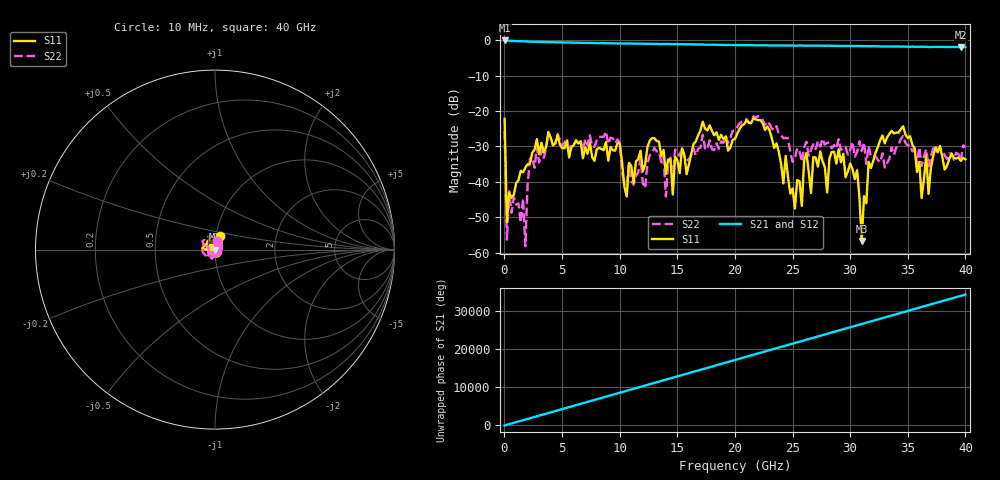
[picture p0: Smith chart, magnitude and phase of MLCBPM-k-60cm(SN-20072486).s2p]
!Keysight Technologies,N5225A,MY51451228,A.10.40.14
!Date: Friday, November 20, 2020 11:33:09
!Correction: S11(Full 2 Port(1,2))
!S21(Full 2 Port(1,2))
!S12(Full 2 Port(1,2))
!S22(Full 2 Port(1,2))
!S2P File: Measurements: S11, S21, S12, S22:
# Hz S  dB  R 50
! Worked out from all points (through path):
!   201 points, 10 MHz to 40 GHz, reference 50 ohm
!   highest |S21| = -0.11 dB at 10 MHz (marker M1); lowest = -2.0 dB at 39.6 GHz (marker M2)
!   lowest |S11| = -56.7 dB at 31 GHz (marker M3), VSWR 1.00, Z = 49.9 + j0.0273 ohm
!   |S11| at or under -10 dB: start of sweep to end of sweep
!   |S22| runs from -58.1 to -21.5 dB; largest |S21 - S12| = 0.0073
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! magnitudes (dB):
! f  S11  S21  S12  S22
! 10 MHz  -22.2  -0.1  -0.1  -25.8
! 209.9 MHz  -51.3  -0.1  -0.1  -56.3
! 409.9 MHz  -43.1  -0.2  -0.2  -42.6
! 1.81 GHz  -35.9  -0.4  -0.4  -58.1
! 2.209 GHz  -34.9  -0.4  -0.4  -33.5
! 2.809 GHz  -27.9  -0.5  -0.5  -30.2
! 6.808 GHz  -33.3  -0.8  -0.8  -31.3
! 10.01 GHz  -29.1  -0.9  -0.9  -29.0
! 10.61 GHz  -44.1  -1.0  -1.0  -40.5
! 13.41 GHz  -28.6  -1.1  -1.1  -31.4
! 14.61 GHz  -43.5  -1.1  -1.1  -39.4
! 20 GHz  -27.9  -1.4  -1.4  -25.5
! 22.8 GHz  -24.4  -1.5  -1.5  -22.9
! 25.2 GHz  -47.5  -1.5  -1.5  -33.2
! 26.8 GHz  -33.0  -1.6  -1.6  -29.4
! 30.6 GHz  -36.7  -1.7  -1.6  -31.5
! 31 GHz  -56.7  -1.7  -1.7  -31.3
! 31.6 GHz  -34.3  -1.7  -1.7  -29.9
! 33.4 GHz  -26.5  -1.8  -1.8  -33.4
! 36.2 GHz  -44.6  -1.9  -1.9  -35.5
! 39.6 GHz  -34.0  -2.0  -2.0  -34.0
! 40 GHz  -33.6  -2.0  -2.0  -30.2
